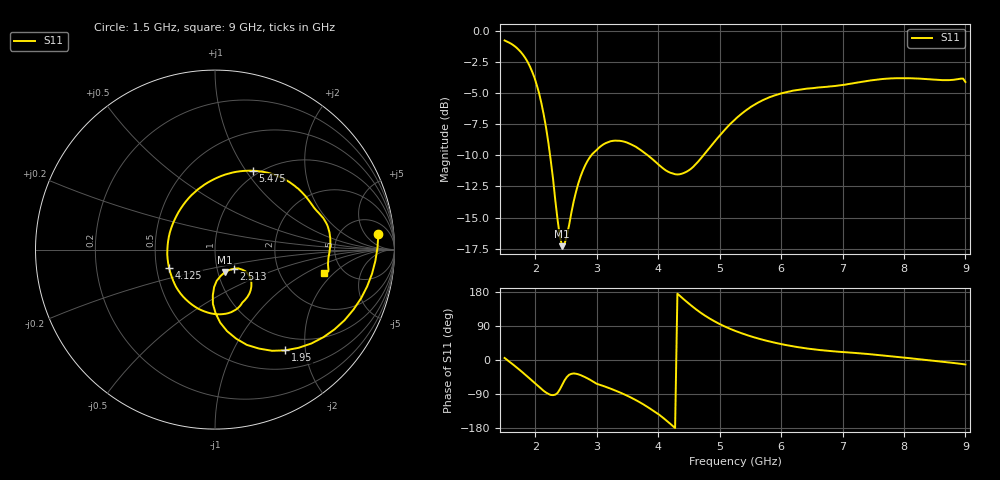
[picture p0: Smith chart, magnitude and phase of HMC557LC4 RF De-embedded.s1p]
! Hittite Microwave Corporation
! 20 Alpha Road
! Chelmsford, MA 01824
! http://www.hittite.com
! Tel: 978-250-3343
! Fax: 978-250-3373
! Device:  HMC557LC4
! Description: GaAS MMIC Fundamental Mixer
! Frequency:  2.5 -  7.0 GHz
! Package:  LC4  - Ceramic- 24 pins
! Ports:  1,RF Port De-emdded from 1.5-9 GHz @-10 dBm , LO FREQ=6GHz @ 15dBm , IF Terminated
! Data:  The device was measured on evaluation board 118703.
!  The evaluation circuit board was modeled and simulated.  This was use
!  to removed the evaluation board circuit from the measured data.
!  The reference plane is the center of the package pin.
! Misc:
! Date Measured:  20-02-2008
! Date:  21-02-2008
! Note:
!  Hittite supplies this data as a sample of measured data at the package pin for
!  for this package product.  Your particular data for this product may vary.
!  Data was taken at 25 degrees C.
!  Hittite reserves the right to change this data at anytime.
# MHz S MA R 50
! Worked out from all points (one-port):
!   201 points, 1.5 GHz to 9 GHz, reference 50 ohm
!   lowest |S11| = -17.3 dB at 2.438 GHz (marker M1), VSWR 1.32, Z = 54.2 - j13.7 ohm
!   |S11| at or under -10 dB: 2.24 GHz to 2.911 GHz (671.6 MHz wide, 26.1 % of centre); 3.831 GHz to 4.736 GHz (904.9 MHz wide, 21.1 % of centre)
!   S11 on the Smith chart (normalised r, x): 1.5 GHz: 11, +11; 1.95 GHz: 0.77, -1.63; 2.513 GHz: 1.21, -0.26; 4.125 GHz: 0.58, -0.13; 5.475 GHz: 0.94, +1.08; 9 GHz: 3.62, -1.52
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1500  0.9142 5.4
1612.5  0.8851 -8.7
1725  0.8406 -23.5
1837.5  0.7767 -38.9
1950  0.6836 -55.2
2062.5  0.5598 -71.5
2175  0.4082 -85.9
2287.5  0.2554 -92.7
2362.5  0.1741 -86.9
2437.5  0.1366 -65.3
2512.5  0.1505 -45.0
2700  0.2442 -37.8
2850  0.3005 -48.6
3075  0.3455 -66.8
3375  0.3616 -85.5
3712.5  0.3324 -112.6
4125  0.2751 -158.6
4312.5  0.265 175.1
4537.5  0.2797 143.7
4800  0.3309 113.2
5250  0.4408 77.1
5475  0.488 64.1
5812.5  0.5413 48.9
6187.5  0.5746 36.3
7125  0.6124 19.6
8062.5  0.6453 5.3
8925  0.6423 -10.1
9000  0.6229 -11.9
